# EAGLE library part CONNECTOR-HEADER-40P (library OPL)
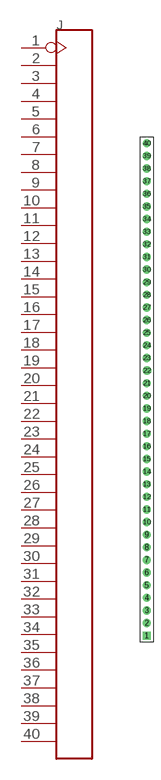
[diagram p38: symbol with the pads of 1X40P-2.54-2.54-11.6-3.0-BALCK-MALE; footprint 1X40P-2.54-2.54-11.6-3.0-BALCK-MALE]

Designator prefix J

## CONNECTOR-HEADER-40P-320020010  [1X40P-2.54-2.54-11.6-3.0-BALCK-MALE]
1  P$1
2  P$2
3  P$3
4  P$4
5  P$5
6  P$6
7  P$7
8  P$8
9  P$9
10  P$10
11  P$11
12  P$12
13  P$13
14  P$14
15  P$15
16  P$16
17  P$17
18  P$18
19  P$19
20  P$20
21  P$21
22  P$22
23  P$23
24  P$24
25  P$25
26  P$26
27  P$27
28  P$28
29  P$29
30  P$30
31  P$31
32  P$32
33  P$33
34  P$34
35  P$35
36  P$36
37  P$37
38  P$38
39  P$39
40  P$40

## Footprint 1X40P-2.54-2.54-11.6-3.0-BALCK-MALE (pad centres in mm)
drill 0.889 pad 1.651 square: 1 0,-49.53
drill 0.889 pad 1.651: 2 0,-46.99; 3 0,-44.45; 4 0,-41.91; 5 0,-39.37; 6 0,-36.83; 7 0,-34.29; 8 0,-31.75; 9 0,-29.21; 10 0,-26.67; 11 0,-24.13; 12 0,-21.59; 13 0,-19.05; 14 0,-16.51; 15 0,-13.97; 16 0,-11.43; 17 0,-8.89; 18 0,-6.35; 19 0,-3.81; 20 0,-1.27; 21 0,1.27; 22 0.025,3.81; 23 0,6.35; 24 0,8.89; 25 0,11.43; 26 0,13.97; 27 0,16.51; 28 0,19.05; 29 0,21.59; 30 0,24.13; 31 0,26.67; 32 0,29.21; 33 0,31.75; 34 0,34.29; 35 0,36.83; 36 0,39.37; 37 0,41.91; 38 0,44.45; 39 0,46.99; 40 0,49.53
